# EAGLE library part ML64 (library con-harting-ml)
HARTING
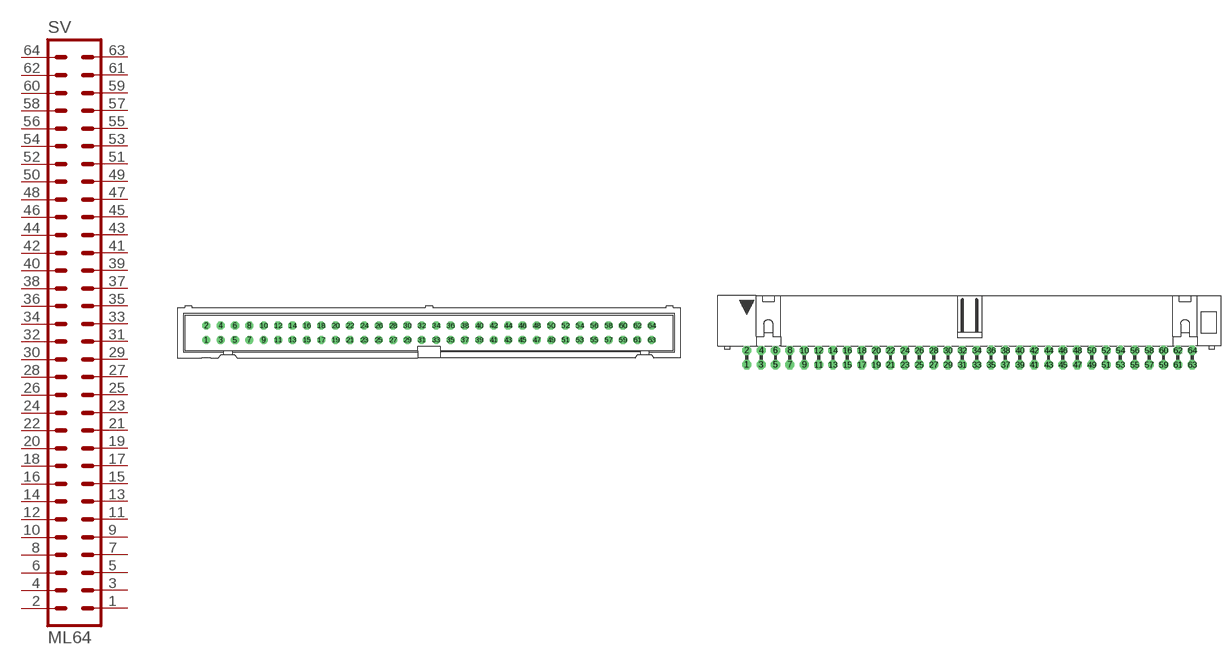
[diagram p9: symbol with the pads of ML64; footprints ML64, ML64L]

Designator prefix SV

## ML64 (OC_FARNELL: unknown; OC_NEWARK: unknown)  [ML64]
1  1  pas
2  2  pas
3  3  pas
4  4  pas
5  5  pas
6  6  pas
7  7  pas
8  8  pas
9  9  pas
10  10  pas
11  11  pas
12  12  pas
13  13  pas
14  14  pas
15  15  pas
16  16  pas
17  17  pas
18  18  pas
19  19  pas
20  20  pas
21  21  pas
22  22  pas
23  23  pas
24  24  pas
25  25  pas
26  26  pas
27  27  pas
28  28  pas
29  29  pas
30  30  pas
31  31  pas
32  32  pas
33  33  pas
34  34  pas
35  35  pas
36  36  pas
37  37  pas
38  38  pas
39  39  pas
40  40  pas
41  41  pas
42  42  pas
43  43  pas
44  44  pas
45  45  pas
46  46  pas
47  47  pas
48  48  pas
49  49  pas
50  50  pas
51  51  pas
52  52  pas
53  53  pas
54  54  pas
55  55  pas
56  56  pas
57  57  pas
58  58  pas
59  59  pas
60  60  pas
61  61  pas
62  62  pas
63  63  pas
64  64  pas

## ML64L (OC_FARNELL: unknown; OC_NEWARK: unknown)  [ML64L]
Pads as for ML64

## ML643M (OC_FARNELL: unknown; OC_NEWARK: unknown)  [3M_64]
Pads as for ML64

## ML643ML (OC_FARNELL: unknown; OC_NEWARK: unknown)  [3M_64L]
Pads as for ML64

## Footprint ML64 (pad centres in mm)
HARTING
drill 0.914 octagon: 1 -39.37,-1.27; 2 -39.37,1.27; 3 -36.83,-1.27; 4 -36.83,1.27; 5 -34.29,-1.27; 6 -34.29,1.27; 7 -31.75,-1.27; 8 -31.75,1.27; 9 -29.21,-1.27; 10 -29.21,1.27; 11 -26.67,-1.27; 12 -26.67,1.27; 13 -24.13,-1.27; 14 -24.13,1.27; 15 -21.59,-1.27; 16 -21.59,1.27; 17 -19.05,-1.27; 18 -19.05,1.27; 19 -16.51,-1.27; 20 -16.51,1.27; 21 -13.97,-1.27; 22 -13.97,1.27; 23 -11.43,-1.27; 24 -11.43,1.27; 25 -8.89,-1.27; 26 -8.89,1.27; 27 -6.35,-1.27; 28 -6.35,1.27; 29 -3.81,-1.27; 30 -3.81,1.27; 31 -1.27,-1.27; 32 -1.27,1.27; 33 1.27,-1.27; 34 1.27,1.27; 35 3.81,-1.27; 36 3.81,1.27; 37 6.35,-1.27; 38 6.35,1.27; 39 8.89,-1.27; 40 8.89,1.27; 41 11.43,-1.27; 42 11.43,1.27; 43 13.97,-1.27; 44 13.97,1.27; 45 16.51,-1.27; 46 16.51,1.27; 47 19.05,-1.27; 48 19.05,1.27; 49 21.59,-1.27; 50 21.59,1.27; 51 24.13,-1.27; 52 24.13,1.27; 53 26.67,-1.27; 54 26.67,1.27; 55 29.21,-1.27; 56 29.21,1.27; 57 31.75,-1.27; 58 31.75,1.27; 59 34.29,-1.27; 60 34.29,1.27; 61 36.83,-1.27; 62 36.83,1.27; 63 39.37,-1.27; 64 39.37,1.27

## Footprint ML64L (pad centres in mm)
HARTING
drill 0.914 pad 1.6 octagon: 1 -39.37,-1.27; 2 -39.37,1.27; 3 -36.83,-1.27; 4 -36.83,1.27; 5 -34.29,-1.27; 6 -34.29,1.27; 7 -31.75,-1.27; 8 -31.75,1.27; 9 -29.21,-1.27; 10 -29.21,1.27; 11 -26.67,-1.27; 12 -26.67,1.27; 13 -24.13,-1.27; 14 -24.13,1.27; 15 -21.59,-1.27; 16 -21.59,1.27; 17 -19.05,-1.27; 18 -19.05,1.27; 19 -16.51,-1.27; 20 -16.51,1.27; 21 -13.97,-1.27; 22 -13.97,1.27; 23 -11.43,-1.27; 24 -11.43,1.27; 25 -8.89,-1.27; 26 -8.89,1.27; 27 -6.35,-1.27; 28 -6.35,1.27; 29 -3.81,-1.27; 30 -3.81,1.27; 31 -1.27,-1.27; 32 -1.27,1.27; 33 1.27,-1.27; 34 1.27,1.27; 35 3.81,-1.27; 36 3.81,1.27; 37 6.35,-1.27; 38 6.35,1.27; 39 8.89,-1.27; 40 8.89,1.27; 41 11.43,-1.27; 42 11.43,1.27; 43 13.97,-1.27; 44 13.97,1.27; 45 16.51,-1.27; 46 16.51,1.27; 47 19.05,-1.27; 48 19.05,1.27; 49 21.59,-1.27; 50 21.59,1.27; 51 24.13,-1.27; 52 24.13,1.27; 53 26.67,-1.27; 54 26.67,1.27; 55 29.21,-1.27; 56 29.21,1.27; 57 31.75,-1.27; 58 31.75,1.27; 59 34.29,-1.27; 60 34.29,1.27; 61 36.83,-1.27; 62 36.83,1.27; 63 39.37,-1.27; 64 39.37,1.27

## Footprint 3M_64 (pad centres in mm)
3M
drill 0.813 square: 1 -39.37,-1.27; 2 -39.37,1.27; 3 -36.83,-1.27; 4 -36.83,1.27; 5 -34.29,-1.27; 6 -34.29,1.27; 7 -31.75,-1.27; 8 -31.75,1.27; 9 -29.21,-1.27; 10 -29.21,1.27; 11 -26.67,-1.27; 12 -26.67,1.27; 13 -24.13,-1.27; 14 -24.13,1.27; 15 -21.59,-1.27; 16 -21.59,1.27; 17 -19.05,-1.27; 18 -19.05,1.27; 19 -16.51,-1.27; 20 -16.51,1.27; 21 -13.97,-1.27; 22 -13.97,1.27; 23 -11.43,-1.27; 24 -11.43,1.27; 25 -8.89,-1.27; 26 -8.89,1.27; 27 -6.35,-1.27; 28 -6.35,1.27; 29 -3.81,-1.27; 30 -3.81,1.27; 31 -1.27,-1.27; 32 -1.27,1.27; 33 1.27,-1.27; 34 1.27,1.27; 35 3.81,-1.27; 36 3.81,1.27; 37 6.35,-1.27; 38 6.35,1.27; 39 8.89,-1.27; 40 8.89,1.27; 41 11.43,-1.27; 42 11.43,1.27; 43 13.97,-1.27; 44 13.97,1.27; 45 16.51,-1.27; 46 16.51,1.27; 47 19.05,-1.27; 48 19.05,1.27; 49 21.59,-1.27; 50 21.59,1.27; 51 24.13,-1.27; 52 24.13,1.27; 53 26.67,-1.27; 54 26.67,1.27; 55 29.21,-1.27; 56 29.21,1.27; 57 31.75,-1.27; 58 31.75,1.27; 59 34.29,-1.27; 60 34.29,1.27; 61 36.83,-1.27; 62 36.83,1.27; 63 39.37,-1.27; 64 39.37,1.27

## Footprint 3M_64L (pad centres in mm)
3M
drill 0.813 square: 1 -39.37,-5.08; 2 -39.37,-2.54; 3 -36.83,-5.08; 4 -36.83,-2.54; 5 -34.29,-5.08; 6 -34.29,-2.54; 7 -31.75,-5.08; 8 -31.75,-2.54; 9 -29.21,-5.08; 10 -29.21,-2.54; 11 -26.67,-5.08; 12 -26.67,-2.54; 13 -24.13,-5.08; 14 -24.13,-2.54; 15 -21.59,-5.08; 16 -21.59,-2.54; 17 -19.05,-5.08; 18 -19.05,-2.54; 19 -16.51,-5.08; 20 -16.51,-2.54; 21 -13.97,-5.08; 22 -13.97,-2.54; 23 -11.43,-5.08; 24 -11.43,-2.54; 25 -8.89,-5.08; 26 -8.89,-2.54; 27 -6.35,-5.08; 28 -6.35,-2.54; 29 -3.81,-5.08; 30 -3.81,-2.54; 31 -1.27,-5.08; 32 -1.27,-2.54; 33 1.27,-5.08; 34 1.27,-2.54; 35 3.81,-5.08; 36 3.81,-2.54; 37 6.35,-5.08; 38 6.35,-2.54; 39 8.89,-5.08; 40 8.89,-2.54; 41 11.43,-5.08; 42 11.43,-2.54; 43 13.97,-5.08; 44 13.97,-2.54; 45 16.51,-5.08; 46 16.51,-2.54; 47 19.05,-5.08; 48 19.05,-2.54; 49 21.59,-5.08; 50 21.59,-2.54; 51 24.13,-5.08; 52 24.13,-2.54; 53 26.67,-5.08; 54 26.67,-2.54; 55 29.21,-5.08; 56 29.21,-2.54; 57 31.75,-5.08; 58 31.75,-2.54; 59 34.29,-5.08; 60 34.29,-2.54; 61 36.83,-5.08; 62 36.83,-2.54; 63 39.37,-5.08; 64 39.37,-2.54
hole 2.54 at -45.288,-3.277
hole 2.54 at 45.288,-3.277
